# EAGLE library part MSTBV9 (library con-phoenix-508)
PHOENIX
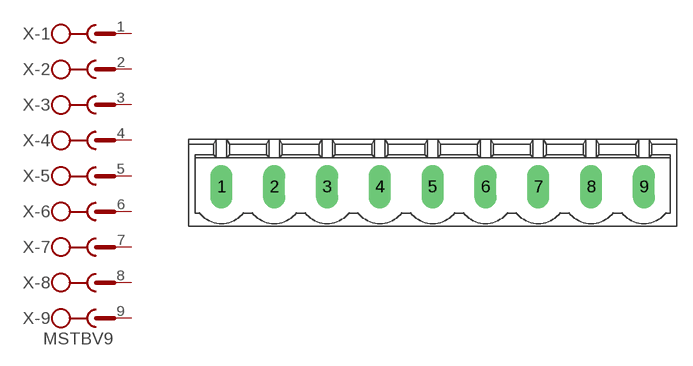
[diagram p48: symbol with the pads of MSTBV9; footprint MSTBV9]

Designator prefix X; gates -1=SK -2=SK -3=SK -4=SK -5=SK -6=SK -7=SK -8=SK -9=SKV

## MSTBV9 (MF: FARNELL; MPN: MSTBVA2,5/9-5,08; OC_FARNELL: 3705328; OC_NEWARK: 71C4149)  [MSTBV9]
1  -1:1  pas
2  -2:1  pas
3  -3:1  pas
4  -4:1  pas
5  -5:1  pas
6  -6:1  pas
7  -7:1  pas
8  -8:1  pas
9  -9:1  pas

## Footprint MSTBV9 (pad centres in mm)
PHOENIX
drill 1.397 long: 1 -20.32,0; 2 -15.24,0; 3 -10.16,0; 4 -5.08,0; 5 0,0; 6 5.08,0; 7 10.16,0; 8 15.24,0; 9 20.32,0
